TYPE ST_Record :
STRUCT
   nID         : ULINT;
   sCustomer   : STRING(50);
   sName       : STRING(50);
   nProductNum : DINT;
   sProductName: STRING(50);
   sProductInfo: T_MaxString;
   tTimestamp  : DT;
END_STRUCT
END_TYPE
